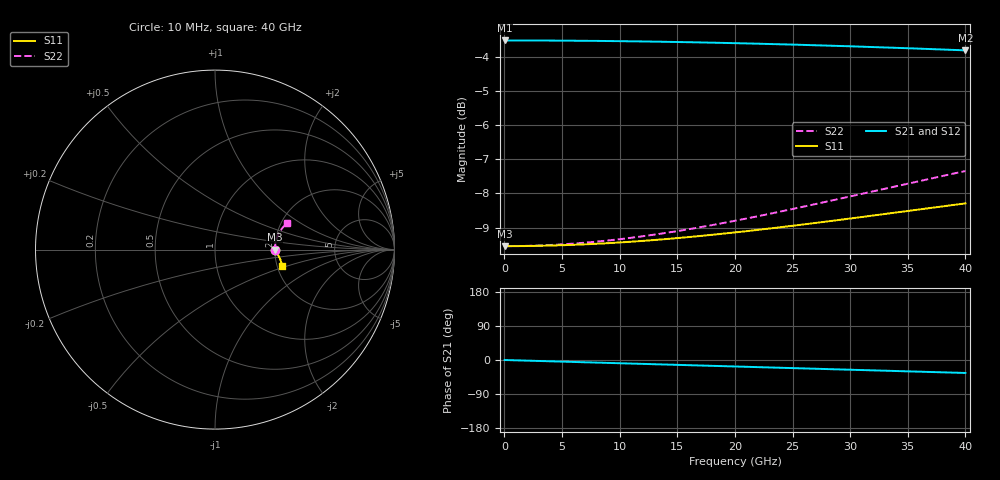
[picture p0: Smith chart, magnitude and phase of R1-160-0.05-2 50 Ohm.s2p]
!version-2
!date-03.2021
# MHz S RI R 50
!Freq ReS11 ImS11 ReS21 ImS21 ReS12 ImS12 ReS22 ImS22
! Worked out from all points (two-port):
!   801 points, 10 MHz to 40 GHz, reference 50 ohm
!   highest |S21| = -3.52 dB at 10 MHz (marker M1); lowest = -3.8 dB at 40 GHz (marker M2)
!   |S21| within 3 dB of the highest: start of sweep to end of sweep
!   lowest |S11| = -9.5 dB at 10 MHz (marker M3), VSWR 2.00, Z = 100 - j0.00188 ohm
!   |S11| at or under -10 dB: nowhere
!   |S22| runs from -9.5 to -7.3 dB; largest |S21 - S12| = 0
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10  0.3333 -8.34e-06  0.6667 -9.99e-05  0.6667 -9.99e-05  0.3333 4.46e-05
210  0.3333 -0.000175  0.6667 -0.0021  0.6667 -0.0021  0.3333 0.000937
1760  0.3335 -0.00147  0.6664 -0.0176  0.6664 -0.0176  0.3335 0.00785
3310  0.3338 -0.0028  0.6657 -0.033  0.6657 -0.033  0.3339 0.0147
5010  0.3344 -0.00431  0.6644 -0.05  0.6644 -0.05  0.3346 0.0223
6710  0.3352 -0.0059  0.6626 -0.0668  0.6626 -0.0668  0.3356 0.0298
8360  0.3362 -0.00757  0.6604 -0.0831  0.6604 -0.0831  0.3369 0.037
10010  0.3374 -0.00937  0.6577 -0.0993  0.6577 -0.0993  0.3384 0.0441
11660  0.3388 -0.0113  0.6545 -0.1155  0.6545 -0.1155  0.3402 0.0512
13360  0.3404 -0.0136  0.6507 -0.1319  0.6507 -0.1319  0.3423 0.0583
15010  0.3422 -0.0159  0.6466 -0.1478  0.6466 -0.1478  0.3446 0.0651
16660  0.344 -0.0186  0.642 -0.1635  0.642 -0.1635  0.3472 0.0719
18310  0.3461 -0.0214  0.6369 -0.179  0.6369 -0.179  0.3499 0.0784
20010  0.3483 -0.0247  0.6313 -0.1948  0.6313 -0.1948  0.353 0.0851
23310  0.3528 -0.032  0.619 -0.2249  0.619 -0.2249  0.3597 0.0974
26710  0.3576 -0.0409  0.6046 -0.2551  0.6046 -0.2551  0.3673 0.1094
30060  0.3624 -0.0513  0.5888 -0.2838  0.5888 -0.2838  0.3755 0.1205
33360  0.3668 -0.0631  0.5718 -0.311  0.5718 -0.311  0.3842 0.1306
35310  0.3692 -0.0709  0.561 -0.3266  0.561 -0.3266  0.3895 0.1361
37260  0.3713 -0.0793  0.5498 -0.3418  0.5498 -0.3418  0.395 0.1414
39760  0.3736 -0.0909  0.5347 -0.3607  0.5347 -0.3607  0.4022 0.1477
40000  0.3738 -0.0921  0.5332 -0.3625  0.5332 -0.3625  0.403 0.1483
